{attribute 'no_assign'}
FUNCTION_BLOCK FB_DO_IED_MUnn_LPHD1_PhyHealth EXTENDS FB_AcsiCommonDataClass
VAR_INPUT
	stVal: FB_AcsiDATypePhyHealth := (Fc:=ACSI_FC_ST, TrgOp:=ACSI_TrgOp_dchg OR ACSI_TrgOp_dupd, bLinkResult:=THIS^.AddDataToContainer(ipData:=stVal));
	q: FB_AcsiDATypeQuality := (Fc:=ACSI_FC_ST, TrgOp:=ACSI_TrgOp_qchg, bLinkResult:=THIS^.AddDataToContainer(ipData:=q));
	t: FB_AcsiDATypeTimeStamp := (Fc:=ACSI_FC_ST, bLinkResult:=THIS^.AddDataToContainer(ipData:=t));
END_VAR
VAR
END_VAR

END_FUNCTION_BLOCK
